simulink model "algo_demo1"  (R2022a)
settings: configuration reference "configurationSettings" (kept in a data dictionary, not in this file)
undefined symbols (not defined in the file or in its folder): algo_demo1_fp, algo_demo1_tp, algo_demo1_tp_build, DiscIntNeverNeededParam, ProductionState, QualityTag, signal1, signal2, signal3, signal4, signal5, signal6, signal7, signal8, signal9, Value

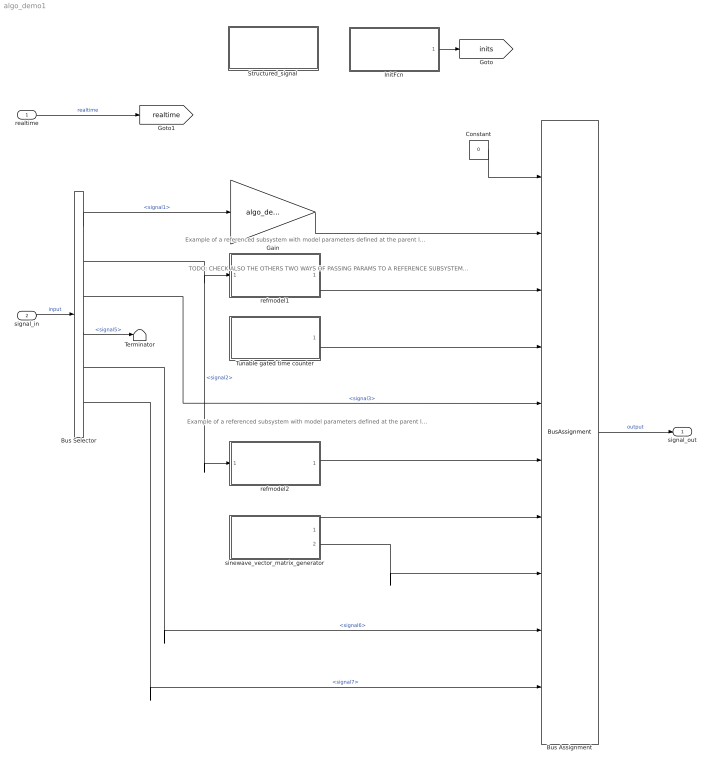
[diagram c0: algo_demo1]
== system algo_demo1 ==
  note: TODO: CHECK ALSO THE OTHERS TWO WAYS OF PASSING PARAMS TO A REFERENCE SUBSYSTEM: 1) VIA MASK (TIMO R REPORTS THAT ONLY SIMULINK.PARAMETER OBJECT CAN BE PASSED) 2) VIA PARAMETER BLOCK FROM THE INIT BLOCK
  note: Example of a referenced subsystem with model parameters defined at the parent level
  note: Example of a referenced subsystem with model parameters defined at the parent level
  realtime : Inport  OutDataTypeStr=single  PortDimensions=1  SampleTime=algo_demo1_fp.timing.dt  Interpolate=off
  signal_in : Inport  Port=2  OutDataTypeStr=Bus: algo_demo1_inBus  PortDimensions=1  Interpolate=off
  Bus Assignment : BusAssignment  AssignedSignals=signal1,signal2,signal3,signal4,signal5,signal6,signal7,signal8,signal9
  Bus Selector : BusSelector  OutputSignals=signal1,signal2,signal3,signal5,signal6,signal7
  Constant : Constant  Value=0  OutDataTypeStr=Bus: algo_demo1_outBus
  Gain : Gain  Gain=algo_demo1_tp.gain
  InitFcn : Subsystem  TreatAsAtomicUnit=on
  Structured_signal : Subsystem  Commented=on
  Terminator : Terminator
  Tunable gated time counter : Subsystem
  refmodel1 : ModelReference  ModelNameDialog=algo_demo1_referenced.slx  UsingDefaultArgumentValue=0,0  SimulationMode=Normal  ModelReferenceVersion=7.0
  refmodel2 : ModelReference  ModelNameDialog=algo_demo1_referenced.slx  UsingDefaultArgumentValue=0,0  SimulationMode=Normal  ModelReferenceVersion=7.0
  sinewave_vector_matrix_generator : Subsystem
  signal_out : Outport  OutDataTypeStr=Bus: algo_demo1_outBus  VectorParamsAs1DForOutWhenUnconnected=off
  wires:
  signal_in/1 -> Bus Selector/1  "input"
  Bus Selector/1 -> Gain/1  "<signal1>"
  Constant/1 -> Bus Assignment/1
  realtime/1 -> [realtime]  "realtime"
  Bus Assignment/1 -> signal_out/1  "output"
  refmodel1/1 -> Bus Assignment/3
  Bus Selector/2 -> refmodel2/1, refmodel1/1  "<signal2>"
  InitFcn/1(InitOut) -> [inits]
  Gain/1 -> Bus Assignment/2
  Tunable gated time counter/1(time) -> Bus Assignment/4
  Bus Selector/3 -> Bus Assignment/5  "<signal3>"
  refmodel2/1 -> Bus Assignment/6
  sinewave_vector_matrix_generator/1(vector_out) -> Bus Assignment/7
  sinewave_vector_matrix_generator/2(matrix_out) -> Bus Assignment/8
  Bus Selector/4 -> Terminator/1  "<signal5>"
  Bus Selector/5 -> Bus Assignment/9  "<signal6>"
  Bus Selector/6 -> Bus Assignment/10  "<signal7>"

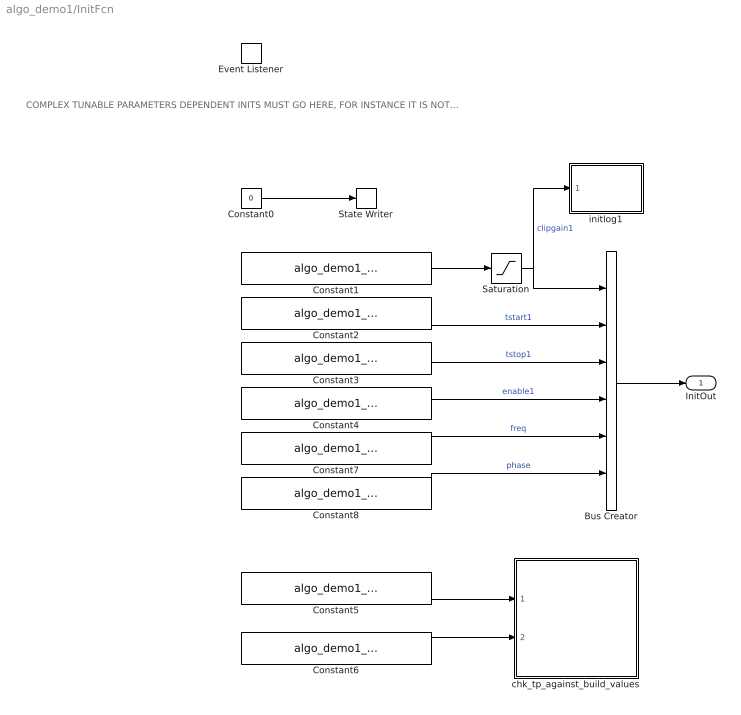
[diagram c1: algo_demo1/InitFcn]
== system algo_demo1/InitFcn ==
  note: COMPLEX TUNABLE PARAMETERS DEPENDENT INITS MUST GO HERE, FOR INSTANCE IT IS NOT POSSIBLE TO REFER TO A TUNABLE PARAMETER VIA DIRECT INDEXING IN MODEL DIALOG, THE VALUE MUST BE EXTRACTED HERE
  Bus Creator : BusCreator  Inputs=6
  Constant0 : Constant  Commented=on  Value=0
  Constant1 : Constant  Value=algo_demo1_tp.gain  OutDataTypeStr=single
  Constant2 : Constant  Value=algo_demo1_tp.colvect(1)  OutDataTypeStr=single
  Constant3 : Constant  Value=algo_demo1_tp.colvect(2)  OutDataTypeStr=single
  Constant4 : Constant  Value=algo_demo1_tp.enable  OutDataTypeStr=boolean
  Constant5 : Constant  Value=algo_demo1_tp  OutDataTypeStr=Bus: algo_demo1_tp_bus
  Constant6 : Constant  Value=algo_demo1_tp_build  OutDataTypeStr=Bus: algo_demo1_tp_bus
  Constant7 : Constant  Value=algo_demo1_tp.colvect(3)  OutDataTypeStr=single
  Constant8 : Constant  Value=algo_demo1_tp.colvect(4)  OutDataTypeStr=single
  Event Listener : EventListener  DisableCoverage=on  EventName=reset
  Saturation : Saturate
  State Writer : StateWriter  Commented=on
  chk_tp_against_build_values : MATLAB Function  TreatAsAtomicUnit=on
  initlog1 : MATLAB Function  TreatAsAtomicUnit=on
  InitOut : Outport  OutDataTypeStr=Bus: algo_demo1_init1  VectorParamsAs1DForOutWhenUnconnected=off
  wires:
  Constant0/1 -> State Writer/1
  Bus Creator/1 -> InitOut/1
  Constant1/1 -> Saturation/1
  Constant2/1 -> Bus Creator/2  "tstart1"
  Saturation/1 -> initlog1/1(u), Bus Creator/1  "clipgain1"
  Constant3/1 -> Bus Creator/3  "tstop1"
  Constant4/1 -> Bus Creator/4  "enable1"
  Constant5/1 -> chk_tp_against_build_values/1(tp)
  Constant6/1 -> chk_tp_against_build_values/2(btp)
  Constant7/1 -> Bus Creator/5  "freq"
  Constant8/1 -> Bus Creator/6  "phase"

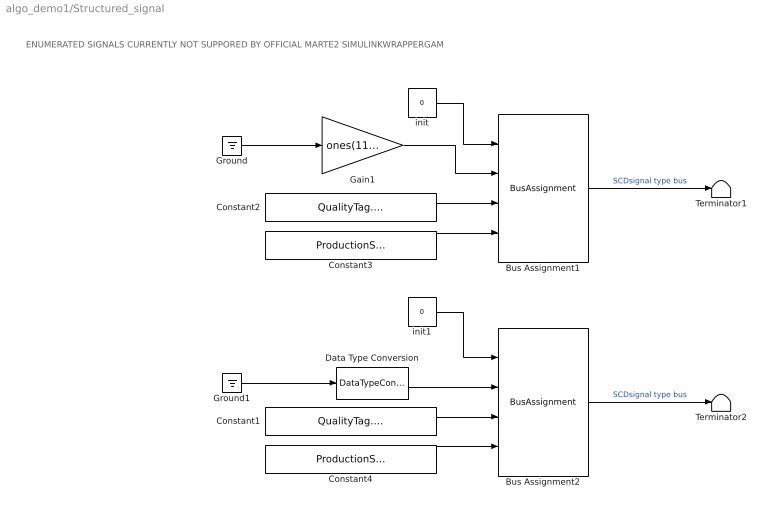
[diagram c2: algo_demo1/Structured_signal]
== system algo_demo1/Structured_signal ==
  note: ENUMERATED SIGNALS CURRENTLY NOT SUPPORED BY OFFICIAL MARTE2 SIMULINKWRAPPERGAM
  Bus Assignment1 : BusAssignment  AssignedSignals=Value,QualityTag,ProductionState
  Bus Assignment2 : BusAssignment  AssignedSignals=Value,QualityTag,ProductionState
  Constant1 : Constant  Value=QualityTag.INVALID  OutDataTypeStr=Enum: QualityTag
  Constant2 : Constant  Value=QualityTag.GOOD  OutDataTypeStr=Enum: QualityTag
  Constant3 : Constant  Value=ProductionState.RUNNING  OutDataTypeStr=Enum: ProductionState
  Constant4 : Constant  Value=ProductionState.OUTDATED  OutDataTypeStr=Enum: ProductionState
  Data Type Conversion : DataTypeConversion  OutDataTypeStr=int32
  Gain1 : Gain  Gain=ones(11,1)
  Ground : Ground
  Ground1 : Ground
  Terminator1 : Terminator
  Terminator2 : Terminator
  init : Constant  Value=0  OutDataTypeStr=Bus: SCDBus_single_11_Vector
  init1 : Constant  Value=0  OutDataTypeStr=Bus: SCDBus_int32_Scalar
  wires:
  Constant4/1 -> Bus Assignment2/4
  Data Type Conversion/1 -> Bus Assignment2/2
  Ground/1 -> Gain1/1
  Constant1/1 -> Bus Assignment2/3
  init1/1 -> Bus Assignment2/1
  init/1 -> Bus Assignment1/1
  Bus Assignment1/1 -> Terminator1/1  "SCDsignal type bus"
  Bus Assignment2/1 -> Terminator2/1  "SCDsignal type bus"
  Constant2/1 -> Bus Assignment1/3
  Constant3/1 -> Bus Assignment1/4
  Gain1/1 -> Bus Assignment1/2
  Ground1/1 -> Data Type Conversion/1

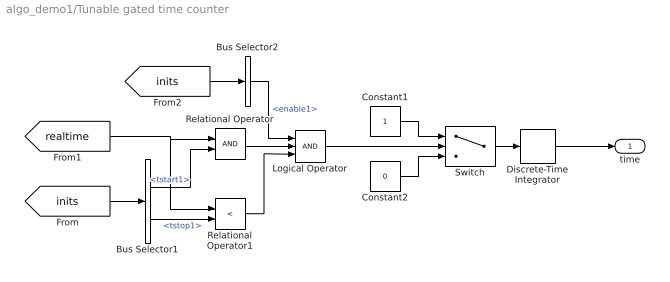
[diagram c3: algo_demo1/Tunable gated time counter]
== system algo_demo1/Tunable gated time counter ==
  Bus Selector1 : BusSelector  OutputSignals=tstart1,tstop1
  Bus Selector2 : BusSelector  OutputSignals=enable1
  Constant1 : Constant  OutDataTypeStr=single
  Constant2 : Constant  Value=0  OutDataTypeStr=single
  Discrete-Time Integrator : DiscreteIntegrator  SampleTime=-1  ICPrevOutput=DiscIntNeverNeededParam  ICPrevScaledInput=DiscIntNeverNeededParam
  Logical Operator : Logic  Inputs=3  AllPortsSameDT=off  OutDataTypeStr=boolean
  Relational Operator : RelationalOperator  OutDataTypeStr=boolean  RndMeth=Simplest
  Relational Operator1 : RelationalOperator  Operator=<  OutDataTypeStr=boolean  RndMeth=Simplest
  Switch : Switch  Criteria=u2 > Threshold
  time : Outport  VectorParamsAs1DForOutWhenUnconnected=off
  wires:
  Bus Selector1/2 -> Relational Operator1/2  "<tstop1>"
  Discrete-Time Integrator/1 -> time/1
  Relational Operator1/1 -> Logical Operator/3
  Bus Selector2/1 -> Logical Operator/1  "<enable1>"
  [inits] -> Bus Selector1/1
  [realtime] -> Relational Operator1/1, Relational Operator/1
  Bus Selector1/1 -> Relational Operator/2  "<tstart1>"
  [inits] -> Bus Selector2/1
  Relational Operator/1 -> Logical Operator/2
  Constant1/1 -> Switch/1
  Constant2/1 -> Switch/3
  Switch/1 -> Discrete-Time Integrator/1
  Logical Operator/1 -> Switch/2

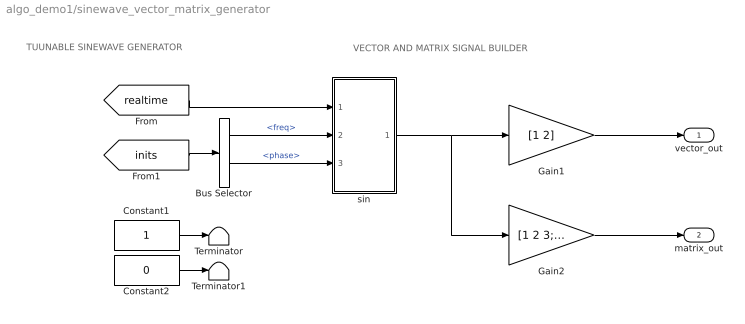
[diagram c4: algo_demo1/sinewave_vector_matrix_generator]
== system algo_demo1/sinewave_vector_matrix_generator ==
  note: TUUNABLE SINEWAVE GENERATOR
  note: VECTOR AND MATRIX SIGNAL BUILDER
  Bus Selector : BusSelector  OutputSignals=freq,phase
  Constant1 : Constant
  Constant2 : Constant  Value=0
  Gain1 : Gain  Gain=[1 2]
  Gain2 : Gain  Gain=[1 2 3; 4 5 6]
  Terminator : Terminator
  Terminator1 : Terminator
  sin : MATLAB Function  TreatAsAtomicUnit=on
  vector_out : Outport  VectorParamsAs1DForOutWhenUnconnected=off
  matrix_out : Outport  Port=2  VectorParamsAs1DForOutWhenUnconnected=off
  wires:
  Gain2/1 -> matrix_out/1
  [realtime] -> sin/1(t)
  Gain1/1 -> vector_out/1
  sin/1(y) -> Gain2/1, Gain1/1
  Constant1/1 -> Terminator/1
  Constant2/1 -> Terminator1/1
  [inits] -> Bus Selector/1
  Bus Selector/1 -> sin/2(f)  "<freq>"
  Bus Selector/2 -> sin/3(ph)  "<phase>"

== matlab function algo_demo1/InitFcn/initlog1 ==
function fcn(u)

fprintf('demo1 tunable gain value is %f\n',u);

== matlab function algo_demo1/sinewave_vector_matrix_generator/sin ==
function y = fcn(t,f,ph)

y = sin(t*2*pi*f+ph);

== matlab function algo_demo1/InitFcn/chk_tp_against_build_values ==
function fcn(tp,btp)

ok=true;

%fields={'enable','gain','rowvect','colvect','matrix','fixdimvector1','fixdimvector2'};

fields=fieldnames(tp);

for i=1:numel(fields)
  if isnumeric(tp.(fields{i}))
    fprintf('chk_tp_against_build_values checking %s',fields{i});
    if ~isequal(tp.(fields{i}),(btp.(fields{i})))
      fprintf(' FAIL.\n');
      ok=false;
    else
      fprintf(' OK.\n');
    end
    fprintf('tp version:\n');
    print3ddata(tp.(fields{i}));
    fprintf('build version:\n');
    print3ddata(btp.(fields{i}));  
  end
end

fprintf('chk_tp_against_build_values ');
if ok
  fprintf('OK.\n');
else
  fprintf('FAIL.\n');
end

end

function print3ddata(M)
  S=int32(size(M));
  if numel(S)<3 
    printmatrix(M);
  elseif numel(S)==3
    for m=1:S(3)
      fprintf("m %d\n",m);
      printmatrix(M(:,:,m))
    end
  end
end

function printmatrix(M)
  S=int32(size(M));
  if numel(S)<3
  for r=1:S(1)
    for c=1:S(2)
      if(isinteger(M(r,c)))
        fprintf("%6d",M(r,c))
      end
      if(isfloat(M(r,c)))
        fprintf("%6.2f ",M(r,c));
      end
    end
    fprintf('\n');
  end
  end
end
